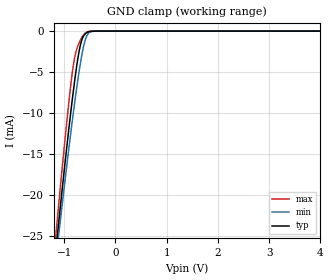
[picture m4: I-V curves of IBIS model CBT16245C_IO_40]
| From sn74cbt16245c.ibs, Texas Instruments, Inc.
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[Model]   CBT16245C_IO_40
Model_type  Terminator
| variable   typ   min   max
C_comp   5.91pF   4.41pF   11.04pF
| C_tri-state   5.91pF   4.41pF   11.04pF
[Temperature Range]   40   100   -40
| Ambient temperature   25   85   -40
[Voltage range]   4   4   4
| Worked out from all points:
|   GND clamp passes 1 mA (typ) near -0.65 V on its own axis
[GND Clamp]
| CBT16245C_IO_40
|   Voltage   I(typ)   I(min)   I(max)
-5V       -286.9mA   -267.5mA   -309.2mA
-1.175V   -27.56mA   -28.75mA   -25.86mA
-1.14V    -25.44mA   -26.81mA   -23.51mA
-1.105V   -23.33mA   -24.88mA   -21.17mA
-1.075V   -21.55mA   -23.24mA   -19.19mA
-920mV    -12.64mA   -15mA      -9.438mA
-815mV    -7.1mA     -9.758mA   -4.012mA
-685mV    -1.8mA     -4.052mA   -1.138mA
-610mV    -508.2uA   -1.614mA   -383.4uA
-550mV    -165.1uA   -505.9uA   -102.8uA
-410mV    -5.67uA    -16.28uA   -1.209uA
4V        351.1pA    1.197nA    114.5pA
